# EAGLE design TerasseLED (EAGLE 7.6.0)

## Sheet 1 of 4: Spannungsversorgung + Controller + DALI
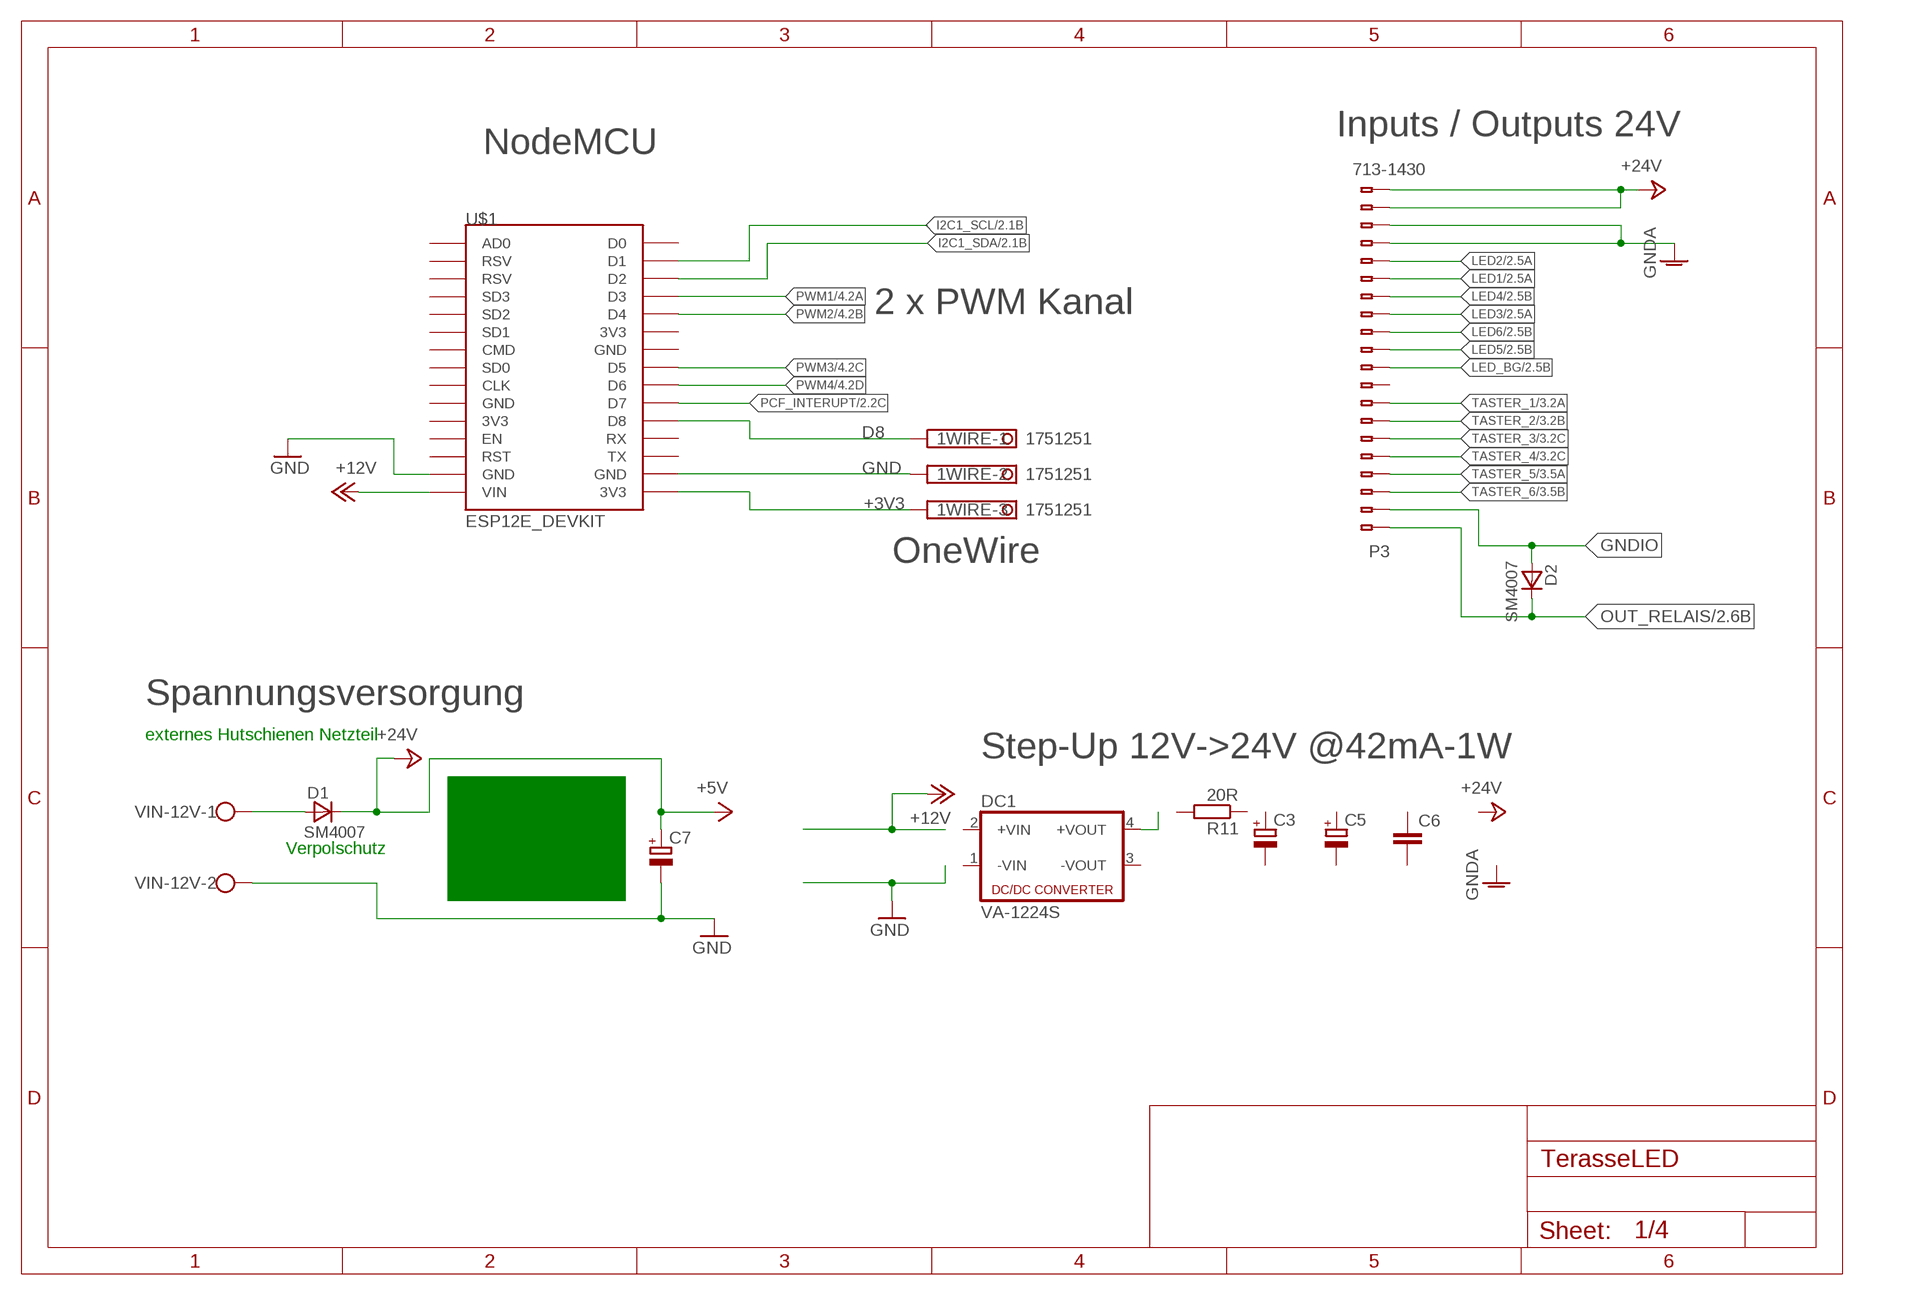
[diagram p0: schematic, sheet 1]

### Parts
1WIRE  1751251  [1751251]
C3  CPOL-EU140CLH-0810  [140CLH-0810]
C5  CPOL-EU140CLH-0810  [140CLH-0810]
C6  C-EUC0805  [C0805]
C7  CPOL-EU140CLH-0810  [140CLH-0810]
D1  SM4007  [MELF-MLL41]
D2  SM4007  [MELF-MLL41]
DC1  VA-1224S  [4SIL]
P3  713-1430  [713-1425]
R11  20R  R-EU_R1206  [R1206]
U$1  ESP12E_DEVKIT  [ESP12E_DEVKIT]
VIN-12V  W237-102  [W237-102]

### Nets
+3V3: 1WIRE.3 U$1.3V3@2(3V3) ; also sheet 2,3
+12V: U$1.VIN
+24V: C7.+ D1.C P3.19(B-19) P3.20(B-20) ; supply symbol labelled +5V ; also sheet 2
D8: 1WIRE.1 U$1.D8
GND: 1WIRE.2 C7.- U$1.GND@1(GND) U$1.GND@3(GND) VIN-12V.2 ; also sheet 2,3,4
GNDA: P3.17(B-17) P3.18(B-18) ; also sheet 2
GNDIO: D2.A P3.2(B-2) ; also sheet 2,3
I2C1_SCL: U$1.D1 ; also sheet 2
I2C1_SDA: U$1.D2 ; also sheet 2
LED1: P3.15(B-15) ; also sheet 2
LED2: P3.16(B-16) ; also sheet 2
LED3: P3.13(B-13) ; also sheet 2
LED4: P3.14(B-14) ; also sheet 2
LED5: P3.11(B-11) ; also sheet 2
LED6: P3.12(B-12) ; also sheet 2
LED_BG: P3.10(B-10) ; also sheet 2
N$1: D1.A VIN-12V.1
N$2: DC1.4(+VOUT)
OUT_RELAIS: D2.C P3.1(B-1) ; also sheet 2
PCF_INTERUPT: U$1.D7 ; also sheet 2
PWM1: U$1.D3 ; also sheet 4
PWM2: U$1.D4 ; also sheet 4
PWM3: U$1.D5 ; also sheet 4
PWM4: U$1.D6 ; also sheet 4
TASTER_1: P3.8(B-8) ; also sheet 3
TASTER_2: P3.7(B-7) ; also sheet 3
TASTER_3: P3.6(B-6) ; also sheet 3
TASTER_4: P3.5(B-5) ; also sheet 3
TASTER_5: P3.4(B-4) ; also sheet 3
TASTER_6: P3.3(B-3) ; also sheet 3
Unconnected: C3.+ C3.- C5.+ C5.- C6.1 C6.2 DC1.1(-VIN) DC1.2(+VIN) DC1.3(-VOUT) P3.9(B-9) R11.1 R11.2 U$1.3V3@0(3V3) U$1.3V3@1(3V3) U$1.AD0 U$1.CLK U$1.CMD U$1.D0 U$1.EN U$1.GND@0(GND) U$1.GND@2(GND) U$1.RST U$1.RSV@0(RSV) U$1.RSV@1(RSV) U$1.RX U$1.SD0 U$1.SD1 U$1.SD2 U$1.SD3 U$1.TX

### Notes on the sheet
- Inputs / Outputs 24V
- NodeMCU
- 2 x PWM Kanal
- OneWire
- Spannungsversorgung
- externes Hutschienen Netzteil
- Step-Up 12V->24V @42mA-1W
- Verpolschutz

## Sheet 2 of 4: Inputs & Outputs
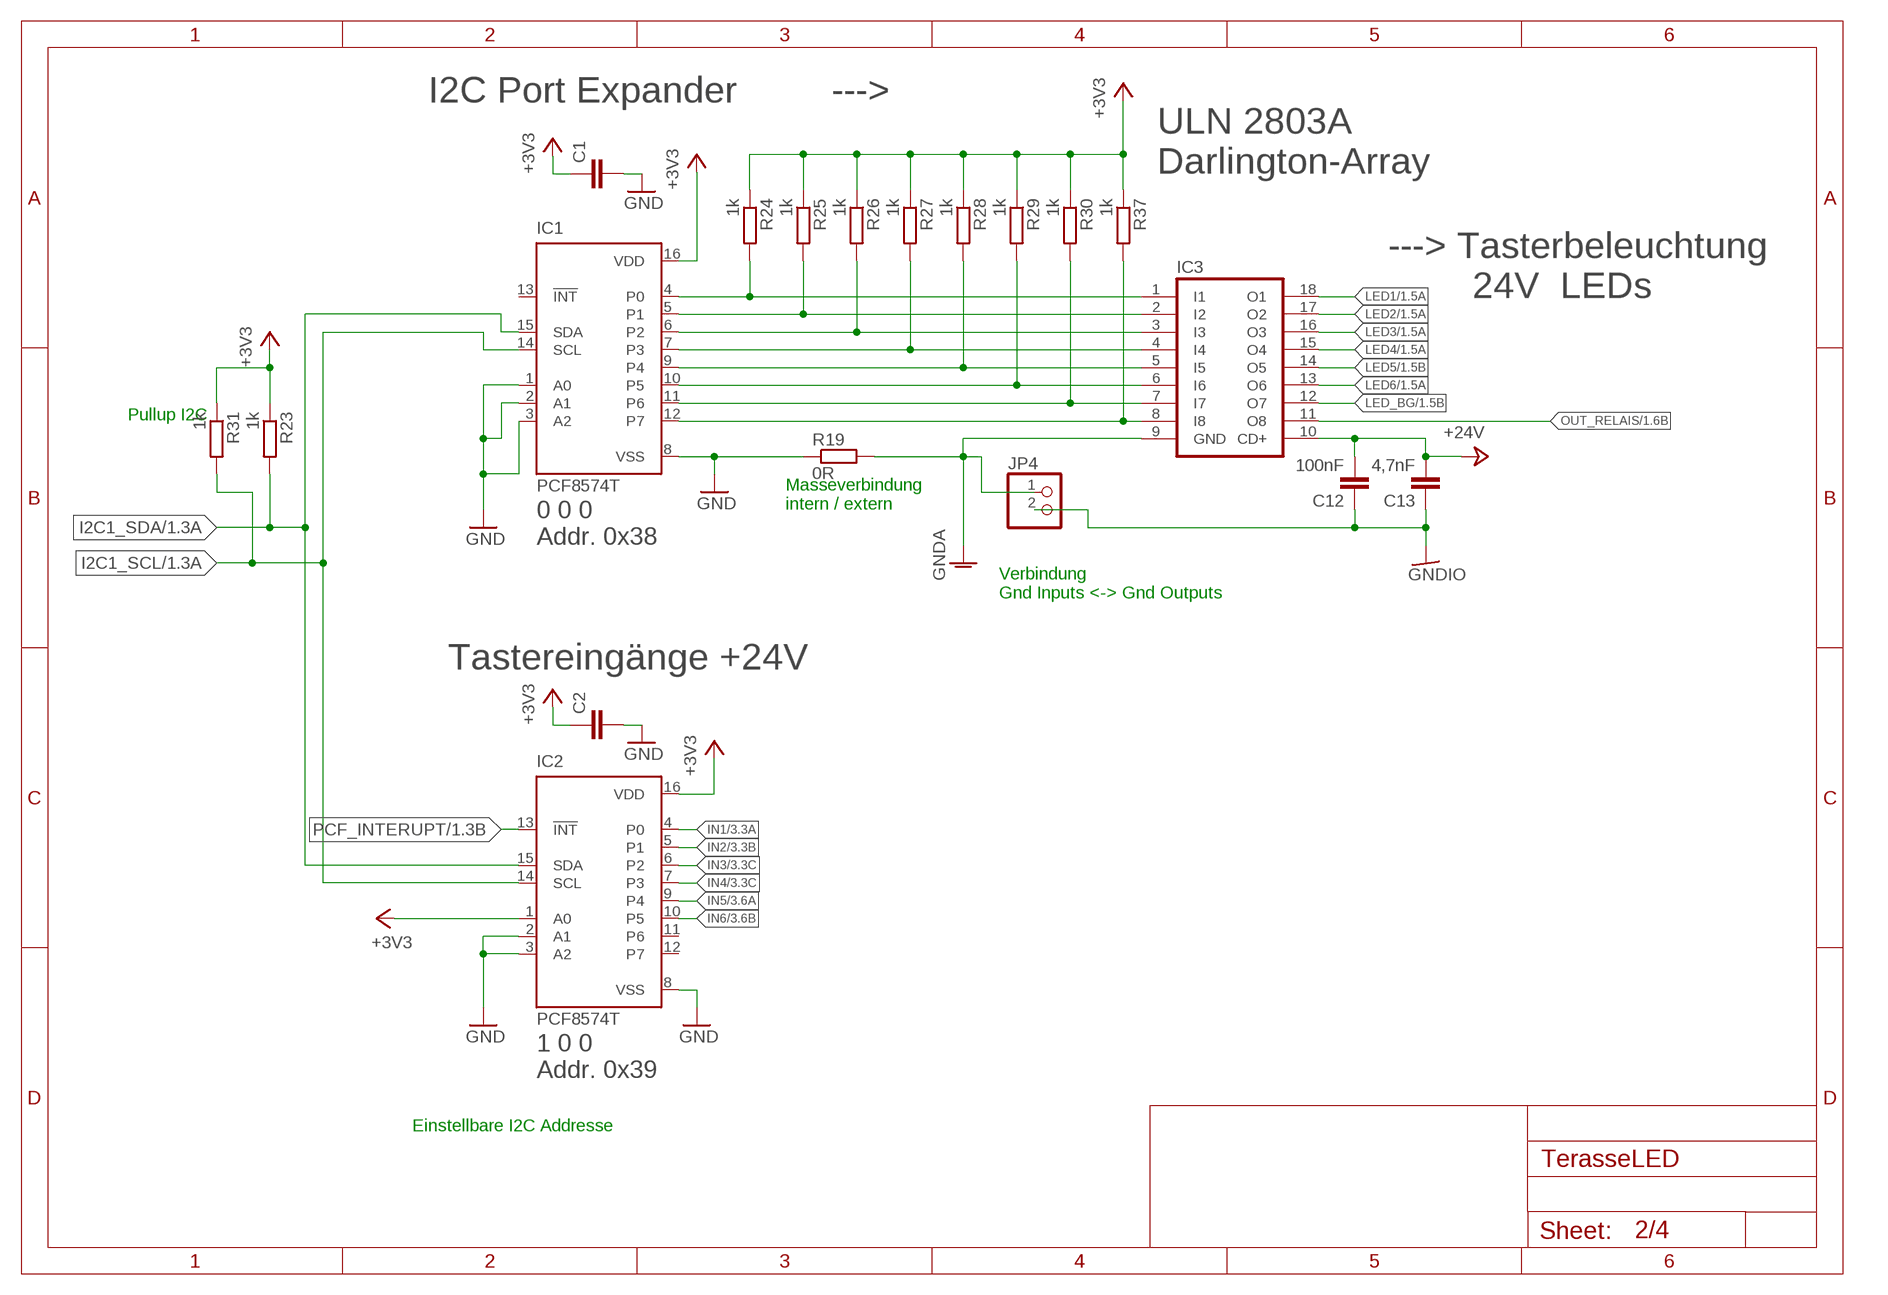
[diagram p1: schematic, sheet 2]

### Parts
C1  C-EUC0805  [C0805]
C2  C-EUC0805  [C0805]
C12  100nF  C-EUC0805  [C0805]
C13  4,7nF  C-EUC0805  [C0805]
IC1  PCF8574T  [SO16W]
IC2  PCF8574T  [SO16W]
IC3  ULN2803ASOP18  [SOP18]
JP4  PINHD-1X2  [1X02]
R19  0R  R-EU_R0805  [R0805]
R23  1k  R-EU_R0805  [R0805]
R24  1k  R-EU_R0805  [R0805]
R25  1k  R-EU_R0805  [R0805]
R26  1k  R-EU_R0805  [R0805]
R27  1k  R-EU_R0805  [R0805]
R28  1k  R-EU_R0805  [R0805]
R29  1k  R-EU_R0805  [R0805]
R30  1k  R-EU_R0805  [R0805]
R31  1k  R-EU_R0805  [R0805]
R37  1k  R-EU_R0805  [R0805]

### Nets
+3V3: C1.1 C2.1 IC1.16(VDD) IC2.1(A0) IC2.16(VDD) R23.1 R24.1 R25.1 R26.1 R27.1 R28.1 R29.1 R30.1 R31.1 R37.1 ; also sheet 1,3
+24V: C12.2 C13.2 IC3.10(CD+) ; also sheet 1
GND: C1.2 C2.2 IC1.1(A0) IC1.2(A1) IC1.3(A2) IC1.8(VSS) IC2.2(A1) IC2.3(A2) IC2.8(VSS) R19.1 ; also sheet 1,3,4
GNDA: IC3.9(GND) JP4.1 R19.2 ; also sheet 1
GNDIO: C12.1 C13.1 JP4.2 ; also sheet 1,3
I2C1_SCL: IC1.14(SCL) IC2.14(SCL) R31.2 ; also sheet 1
I2C1_SDA: IC1.15(SDA) IC2.15(SDA) R23.2 ; also sheet 1
IC1_P0: IC1.4(P0) IC3.1(I1) R24.2
IC1_P1: IC1.5(P1) IC3.2(I2) R25.2
IC1_P2: IC1.6(P2) IC3.3(I3) R26.2
IC1_P3: IC1.7(P3) IC3.4(I4) R27.2
IC1_P4: IC1.9(P4) IC3.5(I5) R28.2
IC1_P5: IC1.10(P5) IC3.6(I6) R29.2
IC1_P6: IC1.11(P6) IC3.7(I7) R30.2
IN1: IC2.4(P0) ; also sheet 3
IN2: IC2.5(P1) ; also sheet 3
IN3: IC2.6(P2) ; also sheet 3
IN4: IC2.7(P3) ; also sheet 3
IN5: IC2.9(P4) ; also sheet 3
IN6: IC2.10(P5) ; also sheet 3
LED1: IC3.18(O1) ; also sheet 1
LED2: IC3.17(O2) ; also sheet 1
LED3: IC3.16(O3) ; also sheet 1
LED4: IC3.15(O4) ; also sheet 1
LED5: IC3.14(O5) ; also sheet 1
LED6: IC3.13(O6) ; also sheet 1
LED_BG: IC3.12(O7) ; also sheet 1
N$19: IC1.12(P7) IC3.8(I8) R37.2
OUT_RELAIS: IC3.11(O8) ; also sheet 1
PCF_INTERUPT: IC2.13(!INT) ; also sheet 1
Unconnected: IC1.13(!INT) IC2.11(P6) IC2.12(P7)

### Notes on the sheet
- I2C Port Expander         --->
- ULN 2803A 
  Darlington-Array
- ---> Tasterbeleuchtung 
          24V  LEDs
- Pullup I2C
- Masseverbindung
  intern / extern
- 0 0 0 
  Addr. 0x38
- Verbindung 
  Gnd Inputs <-> Gnd Outputs
- Tastereingänge +24V
- 1 0 0 
  Addr. 0x39
- Einstellbare I2C Addresse

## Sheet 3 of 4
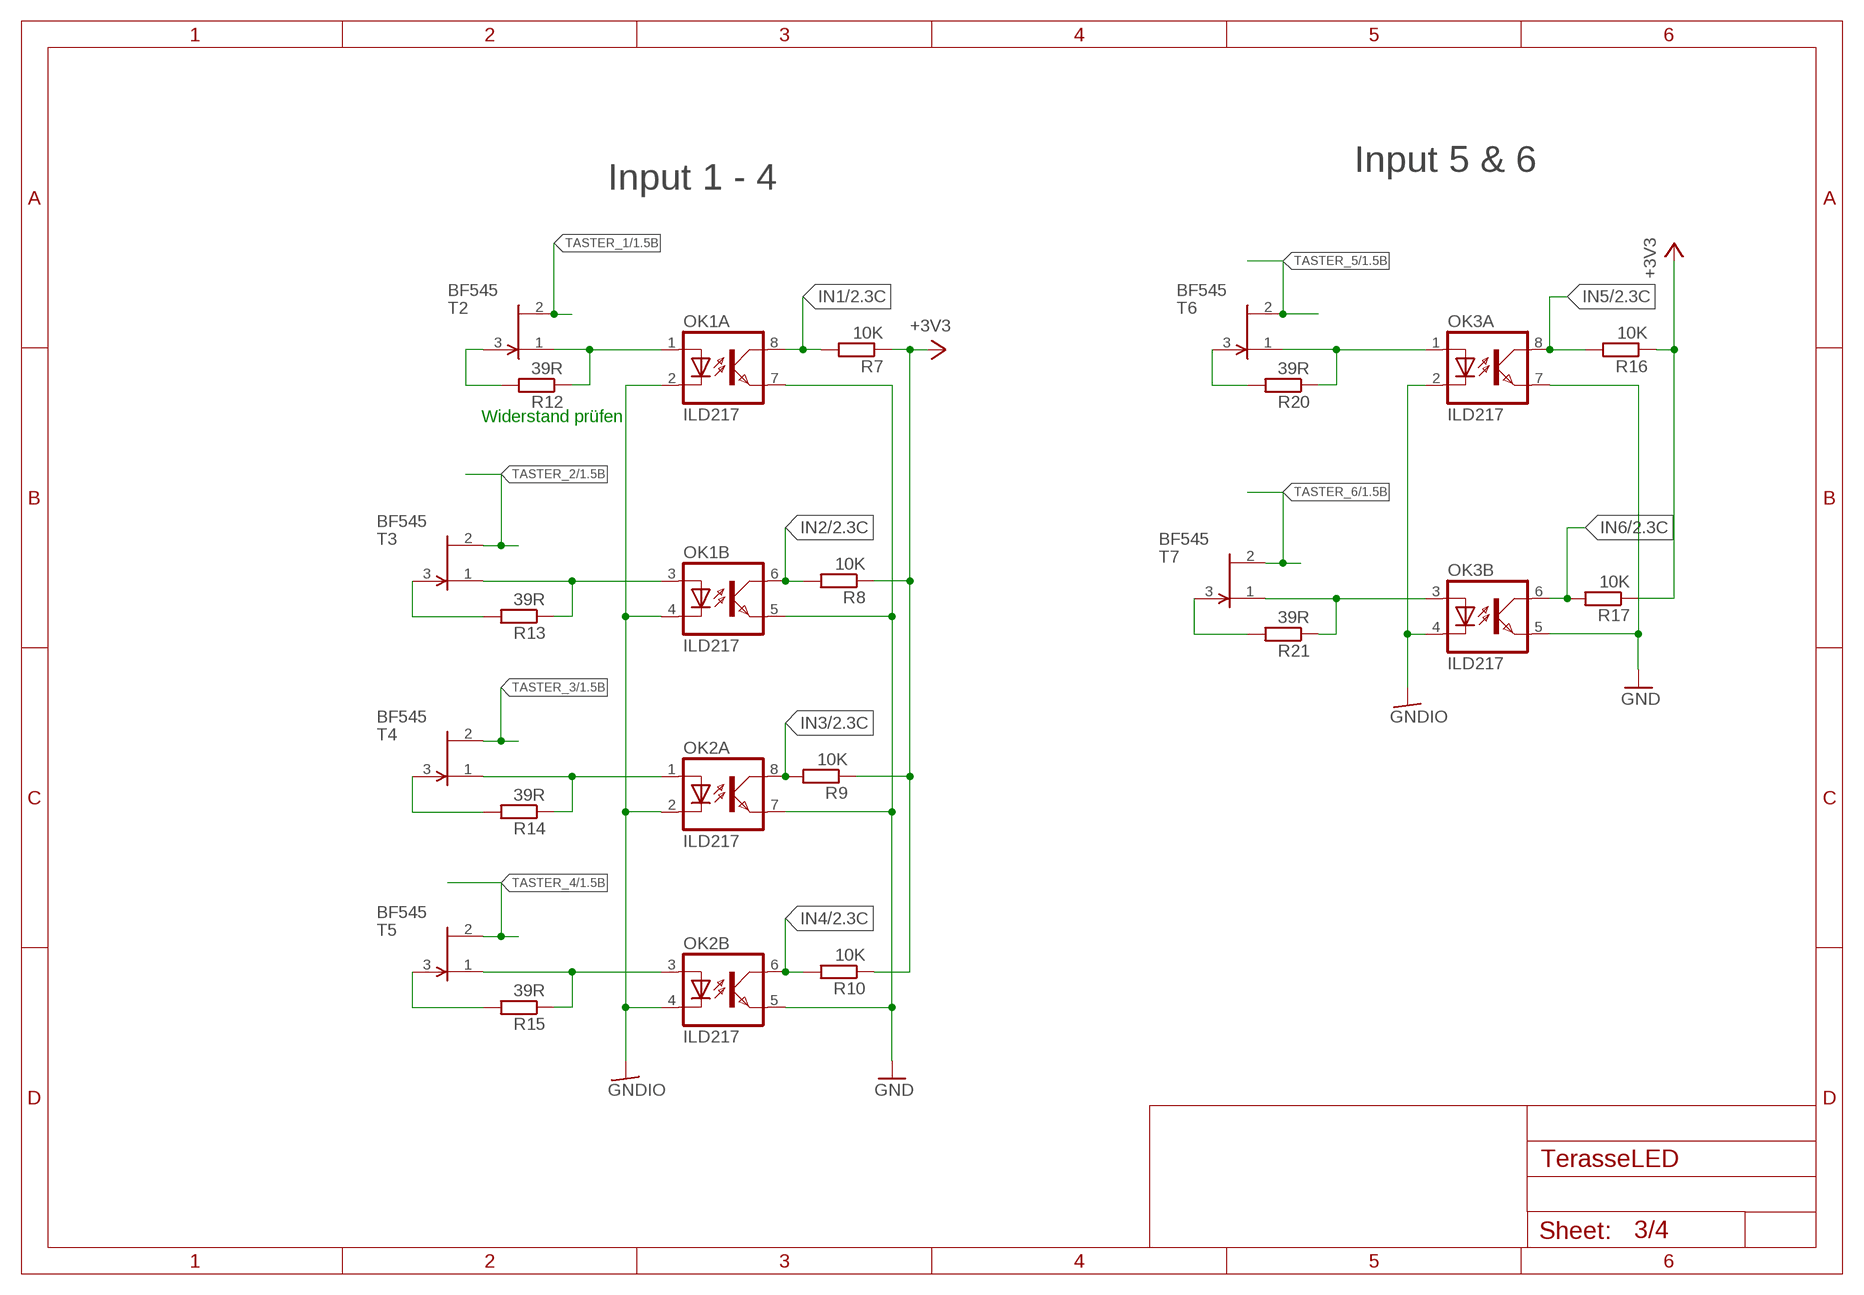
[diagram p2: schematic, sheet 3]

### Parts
OK1  ILD217  [SOIC08]
OK2  ILD217  [SOIC08]
OK3  ILD217  [SOIC08]
R7  10K  R-EU_R0805  [R0805]
R8  10K  R-EU_R0805  [R0805]
R9  10K  R-EU_R0805  [R0805]
R10  10K  R-EU_R0805  [R0805]
R12  39R  R-EU_R0805  [R0805]
R13  39R  R-EU_R0805  [R0805]
R14  39R  R-EU_R0805  [R0805]
R15  39R  R-EU_R0805  [R0805]
R16  10K  R-EU_R0805  [R0805]
R17  10K  R-EU_R0805  [R0805]
R20  39R  R-EU_R0805  [R0805]
R21  39R  R-EU_R0805  [R0805]
T2  BF545  [SOT23]
T3  BF545  [SOT23]
T4  BF545  [SOT23]
T5  BF545  [SOT23]
T6  BF545  [SOT23]
T7  BF545  [SOT23]

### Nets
+3V3: R7.1 R8.1 R9.1 R10.1 R16.1 R17.1 ; also sheet 1,2
GND: OK1.5(B:EMIT) OK1.7(A:EMIT) OK2.5(B:EMIT) OK2.7(A:EMIT) OK3.5(B:EMIT) OK3.7(A:EMIT) ; also sheet 1,2,4
GNDIO: OK1.2(A:C) OK1.4(B:C) OK2.2(A:C) OK2.4(B:C) OK3.2(A:C) OK3.4(B:C) ; also sheet 1,2
IN1: OK1.8(A:COL) R7.2 ; also sheet 2
IN2: OK1.6(B:COL) R8.2 ; also sheet 2
IN3: OK2.8(A:COL) R9.2 ; also sheet 2
IN4: OK2.6(B:COL) R10.2 ; also sheet 2
IN5: OK3.8(A:COL) R16.2 ; also sheet 2
IN6: OK3.6(B:COL) R17.2 ; also sheet 2
N$3: OK2.3(B:A) R15.1 T5.1(S)
N$7: OK2.1(A:A) R14.1 T4.1(S)
N$8: OK1.3(B:A) R13.1 T3.1(S)
N$10: R13.2 T3.3(G)
N$11: R14.2 T4.3(G)
N$12: R15.2 T5.3(G)
N$13: R12.2 T2.3(G)
N$16: OK3.3(B:A) R21.1 T7.1(S)
N$17: R21.2 T7.3(G)
N$20: R20.2 T6.3(G)
Q9_P0_IN: OK1.1(A:A) R12.1 T2.1(S)
Q9_P0_IN1: OK3.1(A:A) R20.1 T6.1(S)
TASTER_1: T2.2(D) ; also sheet 1
TASTER_2: T3.2(D) ; also sheet 1
TASTER_3: T4.2(D) ; also sheet 1
TASTER_4: T5.2(D) ; also sheet 1
TASTER_5: T6.2(D) ; also sheet 1
TASTER_6: T7.2(D) ; also sheet 1

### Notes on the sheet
- Input 5 & 6
- Input 1 - 4
- Widerstand prüfen

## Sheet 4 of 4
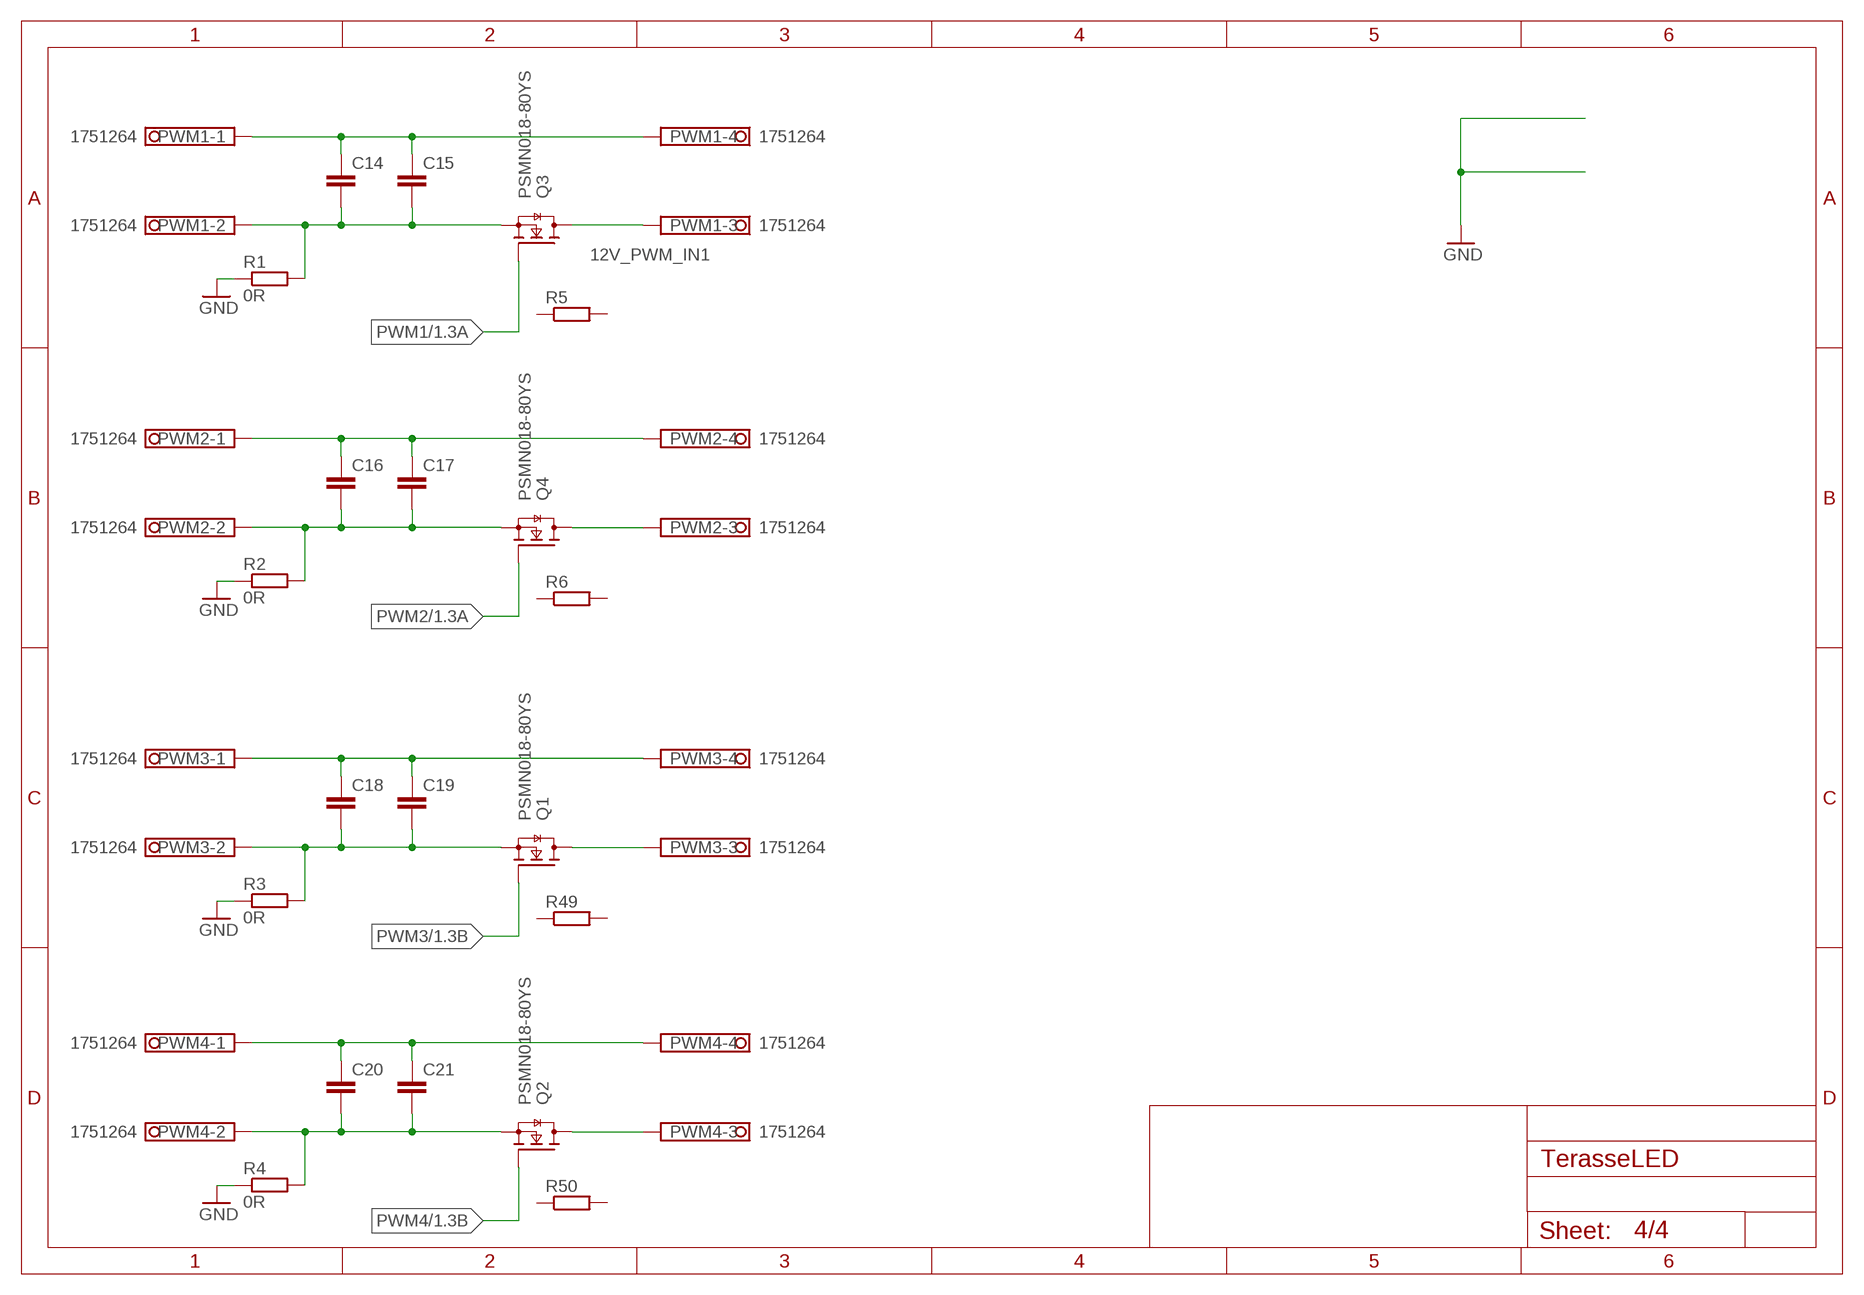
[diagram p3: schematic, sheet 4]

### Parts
C14  C-EUC1206  [C1206]
C15  C-EUC1206  [C1206]
C16  C-EUC1206  [C1206]
C17  C-EUC1206  [C1206]
C18  C-EUC1206  [C1206]
C19  C-EUC1206  [C1206]
C20  C-EUC1206  [C1206]
C21  C-EUC1206  [C1206]
PWM1  1751264  [1751264]
PWM2  1751264  [1751264]
PWM3  1751264  [1751264]
PWM4  1751264  [1751264]
Q1  PSMN018-80YS  [SOT669]
Q2  PSMN018-80YS  [SOT669]
Q3  PSMN018-80YS  [SOT669]
Q4  PSMN018-80YS  [SOT669]
R1  0R  R-EU_R0603  [R0603]
R2  0R  R-EU_R0603  [R0603]
R3  0R  R-EU_R0603  [R0603]
R4  0R  R-EU_R0603  [R0603]
R5  R-EU_R0805  [R0805]
R6  R-EU_R0805  [R0805]
R49  R-EU_R0805  [R0805]
R50  R-EU_R0805  [R0805]

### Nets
12V_PWM_IN1: PWM1.3 Q3.MB(D)
GND: R1.1 R2.1 R3.1 R4.1 ; also sheet 1,2,3
N$4: C14.2 C15.2 PWM1.2 Q3.1(S) Q3.2(S) Q3.3(S) R1.2
N$5: C16.2 C17.2 PWM2.2 Q4.1(S) Q4.2(S) Q4.3(S) R2.2
N$6: C14.1 C15.1 PWM1.1 PWM1.4
N$9: C16.1 C17.1 PWM2.1 PWM2.4
N$21: PWM3.3 Q1.MB(D)
N$25: C18.2 C19.2 PWM3.2 Q1.1(S) Q1.2(S) Q1.3(S) R3.2
N$26: PWM2.3 Q4.MB(D)
N$27: C18.1 C19.1 PWM3.1 PWM3.4
N$28: PWM4.3 Q2.MB(D)
N$29: C20.2 C21.2 PWM4.2 Q2.1(S) Q2.2(S) Q2.3(S) R4.2
N$30: C20.1 C21.1 PWM4.1 PWM4.4
PWM1: Q3.4(G) ; also sheet 1
PWM2: Q4.4(G) ; also sheet 1
PWM3: Q1.4(G) ; also sheet 1
PWM4: Q2.4(G) ; also sheet 1
Unconnected: R5.1 R5.2 R6.1 R6.2 R49.1 R49.2 R50.1 R50.2

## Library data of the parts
1WIRE = con-phoenix-350:1751251: MKDS 1/ 3-3,5 Printklemme Nennstrom: 10 A Bemessungsspannung: 160 V Raster: 3,5 mm Polzahl: 3 Montageart: Löten Anschlussart: Schraubanschluss Anschlussrichtung vom Leiter zur Platine: 0° Source: http://eshop.phoenixcontact.com .. 1751251.pdf; OC_FARNELL: unknown; OC_NEWARK: unknown
C1 C2 C12 C13 = rcl:C-EU: CAPACITOR, European symbol
C3 C5 C7 = resistor:CPOL-EU: POLARIZED CAPACITOR, European symbol
C6 C14-C21 = resistor:C-EU: CAPACITOR, European symbol
D1 D2 = _mod_diode:SM400*: SM4001 .. SM4007 General Purpose Rectifier, 1 A
DC1 = dc-dc-converter:VA-*?: DC DC Converter Single Output, 1 Watt Motien Technology Co.,Ltd. Source: va-serie.pdf
IC1 IC2 = micro-philips:PCF8574: I2C-Bus Remote 8-bit I/O expander http://www.semiconductors.philips.com/acrobat_download/datasheets/PCF8574_4.pdf; MPN: PCF8574T/3,512; OC_FARNELL: 1201255; OC_NEWARK: 70R6870
IC3 = uln-udn:ULN2803A: DRIVER ARRAY
JP4 = pinhead:PINHD-1X2: PIN HEADER
OK1-OK3 = optocoupler:ILD2*: Siemens ILD205/206/207/211/213/217 DUAL PHOTOTRANSISTOR SMALL OUTLINE SURFACE MOUNT OPTOCOUPLER Source: 153385-da-01-en-Optocoupler_ILD205-T.pdf; MF: VISHAY/TELEFUNKEN; MPN: ILD217T; OC_FARNELL: 1469515RL; OC_NEWARK: 20H8681
P3 = con-wago255:713-1430
PWM1-PWM4 = con-phoenix-350:1751264: MKDS 1/ 4-3,5 Printklemme Nennstrom: 10 A Bemessungsspannung: 160 V Raster: 3,5 mm Polzahl: 4 Montageart: Löten Anschlussart: Schraubanschluss Anschlussrichtung vom Leiter zur Platine: 0° Source: http://eshop.phoenixcontact.com .. 1751264.pdf; MPN: 1751264; OC_FARNELL: unknown; OC_NEWARK: 10R0934
Q1-Q4 = NXP_60_26022015:PSMN: N-channel logic level TrenchMOS(TM) transistor AAL Eindhoven MK
R1-R6 R11 R19 R37 R49 R50 = resistor:R-EU_: RESISTOR, European symbol
R7-R10 R12-R17 R20 R21 R23-R31 = rcl:R-EU_: RESISTOR, European symbol
T2-T7 = NXP_60_26022015:BF545
U$1 = ESP12E_DEVKIT:ESP12E_DEVKIT: ESP12E DEVKIT BOARD
VIN-12V = con-wago-500:W237-102: WAGO SCREW CLAMP; MPN: 237-102; OC_FARNELL: unknown; OC_NEWARK: 70K9898

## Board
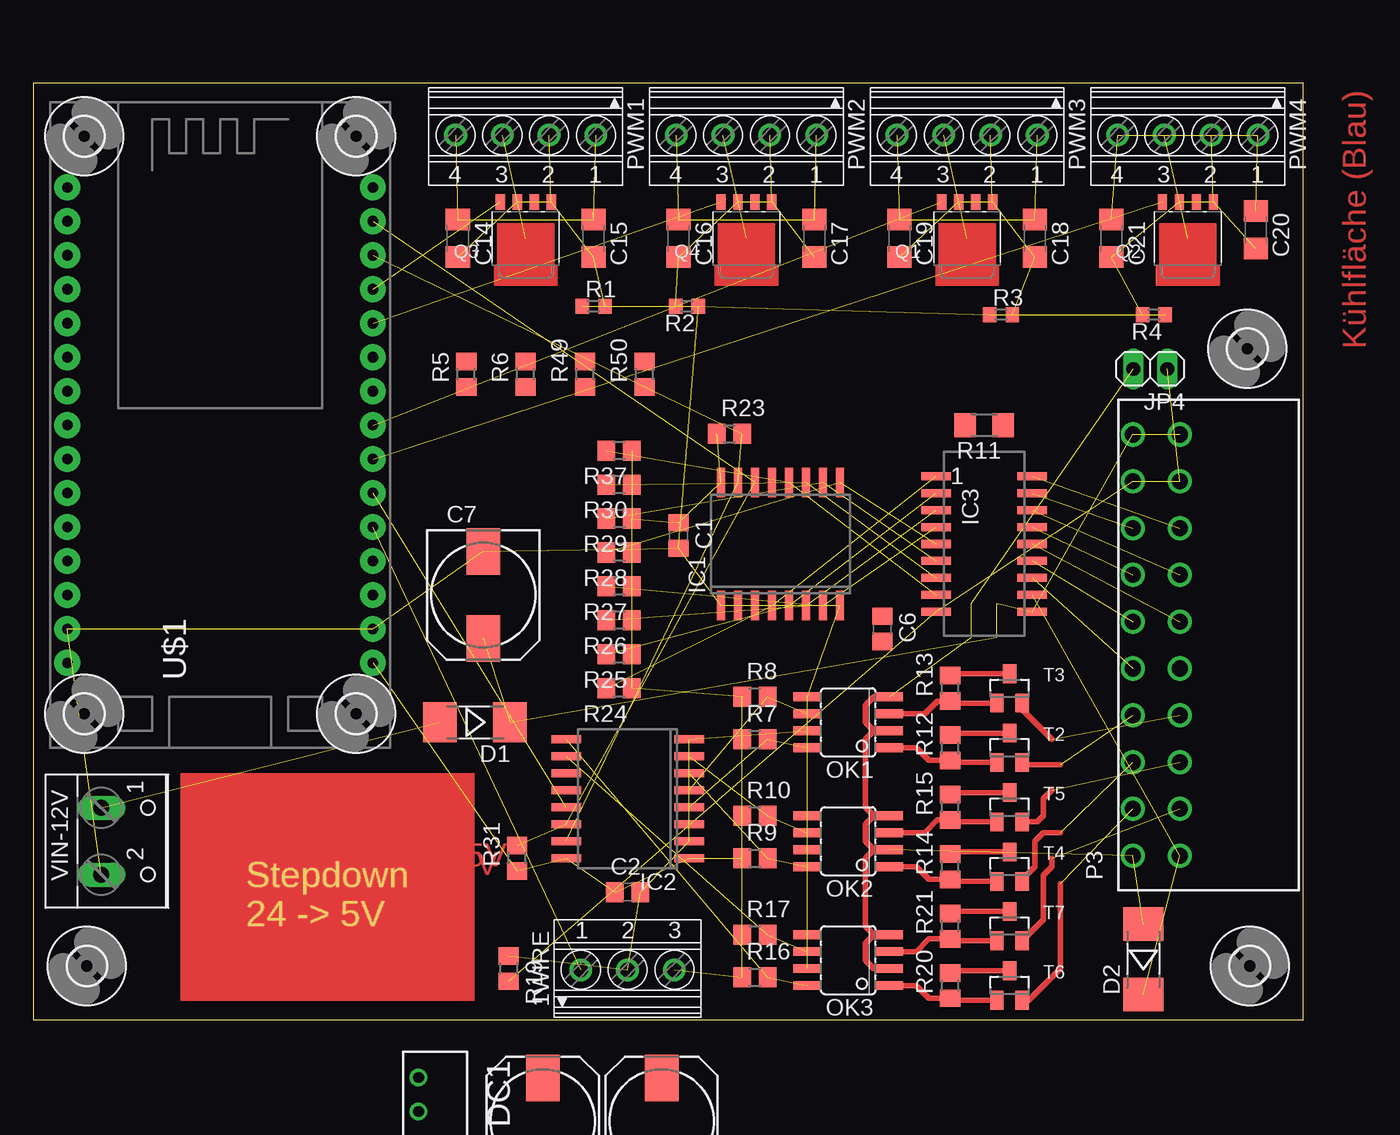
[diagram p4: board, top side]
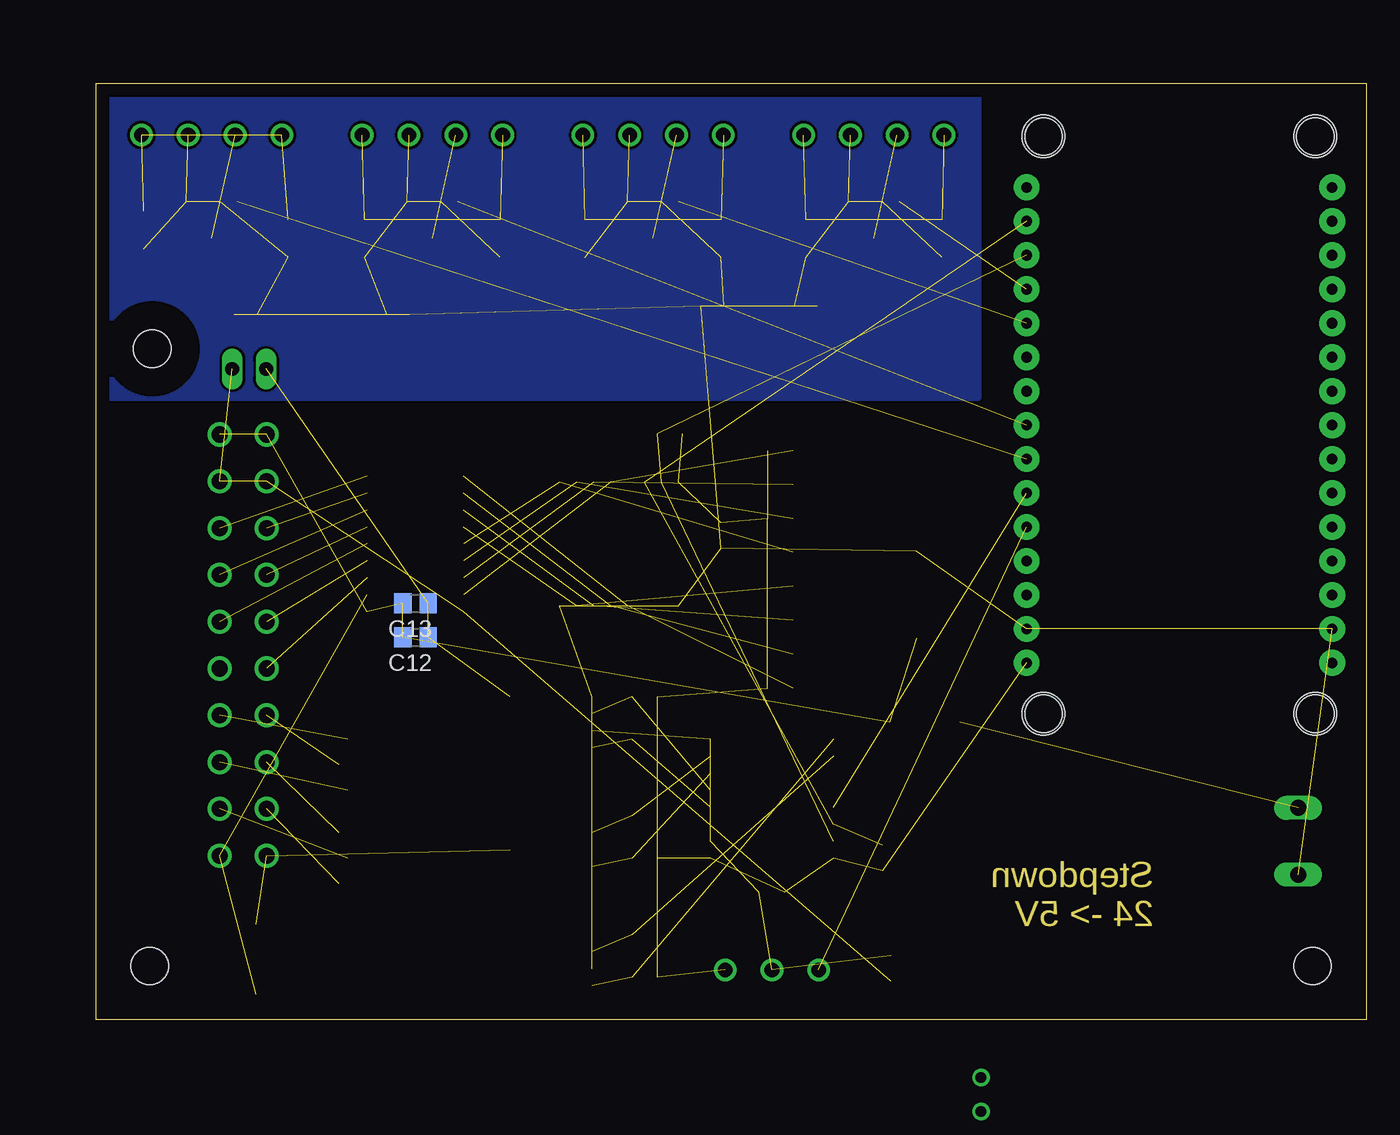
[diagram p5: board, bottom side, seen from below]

Size 95 x 70 mm. Coordinates in mm from the lower left corner, seen from the top.
Outline: 95,0 95,70 0,70 0,0 95,0
Copper layers (1*16): Top 0.035mm / dielectric 1.5mm / Bottom 0.035mm
Design rules "default": minimum track width 10mil, minimum drill 24mil, track to track 8mil, track to pad 8mil, pad to pad 8mil, via to via 8mil, smd to smd 8mil, copper to edge 40mil, drill to drill 8mil, minimum pad ring 10mil, minimum via ring 8mil, stop-mask expansion 4mil, vias tented up to drill 0mil, thermal gap 10mil

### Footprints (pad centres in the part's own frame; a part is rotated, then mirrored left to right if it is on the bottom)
1751251 = drill 1.1 pad 1.7: 1 -3.5,-0.1; 2 0,-0.1; 3 3.5,-0.1
C0805 = smd 1.3 x 1.5: 1 -0.95,0; 2 0.95,0
140CLH-0810 = smd 3.5 x 2.5: + 3.25,0; - -3.25,0
C1206 = smd 1.6 x 1.8: 1 -1.4,0; 2 1.4,0
MELF-MLL41 = smd 2.5 x 3: A 2.625,0; C -2.625,0
4SIL = drill 0.8: 1 -3.81,0; 2 -1.27,0; 3 1.27,0; 4 3.81,0
SO16W = smd 0.6 x 2.2: 1 -4.445,-4.6; 2 -3.175,-4.6; 3 -1.905,-4.6; 4 -0.635,-4.6; 5 0.635,-4.6; 6 1.905,-4.6; 7 3.175,-4.6; 8 4.445,-4.6; 9 4.445,4.6; 10 3.175,4.6; 11 1.905,4.6; 12 0.635,4.6; 13 -0.635,4.6; 14 -1.905,4.6; 15 -3.175,4.6; 16 -4.445,4.6
SOP18 = smd 0.6 x 2.2: 1 -5.08,-3.6; 2 -3.81,-3.6; 3 -2.54,-3.6; 4 -1.27,-3.6; 5 0,-3.6; 6 1.27,-3.6; 7 2.54,-3.6; 8 3.81,-3.6; 9 5.08,-3.6; 10 5.08,3.6; 11 3.81,3.6; 12 2.54,3.6; 13 1.27,3.6; 14 0,3.6; 15 -1.27,3.6; 16 -2.54,3.6; 17 -3.81,3.6; 18 -5.08,3.6
1X02 = drill 1.016 long: 1 -1.27,0; 2 1.27,0
SOIC08 = smd 0.66 x 2.032: 1 -1.905,-3.073; 2 -0.635,-3.073; 3 0.635,-3.073; 4 1.905,-3.073; 5 1.905,3.073; 6 0.635,3.073; 7 -0.635,3.073; 8 -1.905,3.073
713-1425 = drill 1.2: 1 -15.75,-1.75; 2 -15.75,1.75; 3 -12.25,-1.75; 4 -12.25,1.75; 5 -8.75,-1.75; 6 -8.75,1.75; 7 -5.25,-1.75; 8 -5.25,1.75; 9 -1.75,-1.75; 10 -1.75,1.75; 11 1.75,-1.75; 12 1.75,1.75; 13 5.25,-1.75; 14 5.25,1.75; 15 8.75,-1.75; 16 8.75,1.75; 17 12.25,-1.75; 18 12.25,1.75; 19 15.75,-1.75; 20 15.75,1.75
1751264 = drill 1.1 pad 1.7: 1 -5.25,-0.1; 2 -1.75,-0.1; 3 1.75,-0.1; 4 5.25,-0.1
SOT669 = smd 0.7 x 1.15: 1 -1.905,-2.725; 2 -0.636,-2.725; 3 0.635,-2.725; 4 1.905,-2.725 | smd 0 x 0: MB 0,0
R0603 = smd 1 x 1.1: 1 -0.85,0; 2 0.85,0
R0805 = smd 1.3 x 1.5: 1 -0.95,0; 2 0.95,0
R1206 = smd 1.6 x 1.803: 1 -1.422,0; 2 1.422,0
SOT23 = smd 1 x 1.4: 1 -0.95,-1.1; 2 0.95,-1.1; 3 0,1.1
ESP12E_DEVKIT = drill 0.8 pad 1.93: 3V3@0 -11.43,-7.62; 3V3@1 11.43,5.08; 3V3@2 11.43,-17.78; AD0 -11.43,17.78; CLK -11.43,-2.54; CMD -11.43,2.54; D0 11.43,17.78; D1 11.43,15.24; D2 11.43,12.7; D3 11.43,10.16; D4 11.43,7.62; D5 11.43,0; D6 11.43,-2.54; D7 11.43,-5.08; D8 11.43,-7.62; EN -11.43,-10.16; GND@0 -11.43,-5.08; GND@1 -11.43,-15.24; GND@2 11.43,2.54; GND@3 11.43,-15.24; RST -11.43,-12.7; RSV@0 -11.43,15.24; RSV@1 -11.43,12.7; RX 11.43,-10.16; SD0 -11.43,0; SD1 -11.43,5.08; SD2 -11.43,7.62; SD3 -11.43,10.16; TX 11.43,-12.7; VIN -11.43,-17.78 | hole 3.2: -10.16,21.59; 10.16,21.59; 10.16,-21.59; -10.16,-21.59
2,8 = hole 2.8: 0,0
W237-102 = drill 1.194 long: 1 -2.5,-1.27; 2 2.5,-1.27

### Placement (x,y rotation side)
1WIRE  44.45,3.81 0 top
C1  48.26,36.2 270 top
C2  44.45,9.53 0 top
C3  not placed on the board
C5  not placed on the board
C6  63.5,29.21 270 top
C7  33.66,31.75 270 top
C12  71.12,28.57 180 bottom
C13  71.12,31.11 180 bottom
C14  31.75,58.42 270 top
C15  41.91,58.42 270 top
C16  48.26,58.42 270 top
C17  58.42,58.42 270 top
C18  74.93,58.42 270 top
C19  64.77,58.42 270 top
C20  91.44,59.05 270 top
C21  80.64,58.42 270 top
D1  33.02,22.23 180 top
D2  83.03,4.51 90 top
DC1  not placed on the board
IC1  55.88,35.56 0 top
IC2  44.45,16.51 90 top
IC3  71.12,35.56 270 top
JP4  83.56,48.65 180 top
OK1  60.96,22.23 90 top
OK2  60.96,13.34 90 top
OK3  60.96,4.45 90 top
P3  84,28 90 top
PWM1  36.83,66.04 180 top
PWM2  53.34,66.04 180 top
PWM3  69.85,66.04 180 top
PWM4  86.36,66.04 180 top
Q1  69.85,58.42 180 top
Q2  86.36,58.42 180 top
Q3  36.83,58.42 180 top
Q4  53.34,58.42 180 top
R1  41.91,53.34 0 top
R2  48.9,53.34 180 top
R3  72.39,52.7 0 top
R4  83.82,52.7 180 top
R5  32.38,48.26 90 top
R6  36.83,48.26 90 top
R7  53.98,20.95 0 top
R8  53.98,24.13 0 top
R9  53.98,12.06 0 top
R10  53.98,15.24 0 top
R11  71.12,44.45 180 top
R12  68.58,20.32 90 top
R13  68.58,24.77 90 top
R14  68.58,11.43 90 top
R15  68.58,15.88 90 top
R16  53.98,3.17 0 top
R17  53.98,6.35 0 top
R19  35.56,3.81 270 top
R20  68.58,2.54 90 top
R21  68.58,6.99 90 top
R23  52.07,43.81 0 top
R24  43.81,24.77 180 top
R25  43.81,27.3 180 top
R26  43.81,29.84 180 top
R27  43.81,32.38 180 top
R28  43.81,34.92 180 top
R29  43.81,37.47 180 top
R30  43.81,40.01 180 top
R31  36.2,12.06 90 top
R37  43.81,42.55 180 top
R49  41.27,48.26 90 top
R50  45.72,48.26 90 top
T2  73.03,20.32 0 top
T3  73.03,24.77 0 top
T4  73.03,11.43 0 top
T5  73.03,15.88 0 top
T6  73.03,2.54 0 top
T7  73.03,6.99 0 top
U$1  13.97,44.45 0 top
U$2  [2,8]  3.81,66.04 0 top
U$3  [2,8]  3.81,22.86 0 top
U$4  [2,8]  24.13,22.86 0 top
U$5  [2,8]  24.13,66.04 0 top
U$6  [2,8]  90.81,50.16 0 top
U$7  [2,8]  4,4 0 top
U$8  [2,8]  91,4 0 top
VIN-12V  6.35,13.34 270 top

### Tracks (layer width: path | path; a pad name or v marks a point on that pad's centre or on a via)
12V_PWM_IN1  (1 unrouted)
+3V3  (22 unrouted)
+24V  (6 unrouted)
D8  (1 unrouted)
GND  (24 unrouted)
  pour Bottom: 29,46.46 29,69.5 95,69.5 95,46.46
GNDA  (4 unrouted)
GNDIO  (5 unrouted)
  Top 0.406: OK1.4 62.87,24.13 62.23,23.5 62.23,22.23 62.87,21.59 | OK1.2 62.87,21.59 | 62.87,21.59 62.23,20.95 62.23,15.88 62.87,15.24 | OK2.4 62.87,15.24 | 62.87,15.24 62.23,14.61 62.23,13.34 62.87,12.7 | 62.87,12.7 OK2.2 | 62.87,6.35 62.23,6.99 62.23,12.06 62.87,12.7 | OK3.4 62.87,6.35 | 62.87,6.35 62.23,5.71 62.23,4.45 62.87,3.81 OK3.2
I2C1_SCL  (3 unrouted)
I2C1_SDA  (3 unrouted)
IC1_P0  (2 unrouted)
IC1_P1  (2 unrouted)
IC1_P2  (2 unrouted)
IC1_P3  (2 unrouted)
IC1_P4  (2 unrouted)
IC1_P5  (2 unrouted)
IC1_P6  (2 unrouted)
IN1  (2 unrouted)
IN2  (2 unrouted)
IN3  (2 unrouted)
IN4  (2 unrouted)
IN5  (2 unrouted)
IN6  (2 unrouted)
LED1  (1 unrouted)
LED2  (1 unrouted)
LED3  (1 unrouted)
LED4  (1 unrouted)
LED5  (1 unrouted)
LED6  (1 unrouted)
LED_BG  (1 unrouted)
N$1  (1 unrouted)
N$3
  Top 0.406: T5.1 68.73,14.78 R15.1 67.63,14.93 66.67,13.97 OK2.3
N$4  (6 unrouted)
N$5  (6 unrouted)
N$6  (3 unrouted)
N$7
  Top 0.406: T4.1 68.73,10.33 R14.1 66.99,10.48 66.04,11.43 OK2.1
N$8
  Top 0.406: T3.1 68.73,23.66 R13.1 67.63,23.82 66.67,22.86 OK1.3
N$9  (3 unrouted)
N$10
  Top 0.406: T3.3 68.73,25.86 R13.2
N$11
  Top 0.406: T4.3 68.73,12.53 R14.2
N$12
  Top 0.406: T5.3 68.73,16.98 R15.2
N$13
  Top 0.406: T2.3 68.73,21.42 R12.2
N$16
  Top 0.406: T7.1 68.73,5.88 R21.1 67,6.04 66.04,5.08 OK3.3
N$17
  Top 0.406: T7.3 68.73,8.09 R21.2
N$19  (2 unrouted)
N$20
  Top 0.406: T6.3 68.73,3.64 R20.2
N$21  (1 unrouted)
N$25  (6 unrouted)
N$26  (1 unrouted)
N$27  (3 unrouted)
N$28  (1 unrouted)
N$29  (6 unrouted)
N$30  (3 unrouted)
OUT_RELAIS  (2 unrouted)
PCF_INTERUPT  (1 unrouted)
PWM1  (1 unrouted)
PWM2  (1 unrouted)
PWM3  (1 unrouted)
PWM4  (1 unrouted)
Q9_P0_IN
  Top 0.406: T2.1 68.73,19.22 R12.1 66.99,19.37 66.04,20.32 OK1.1
Q9_P0_IN1
  Top 0.406: T6.1 68.73,1.44 R20.1 66.99,1.59 66.04,2.54 OK3.1
TASTER_1  (1 unrouted)
  Top 0.406: 74.12,19.22 T2.2 74.14,19.05 76.83,19.05
TASTER_2  (1 unrouted)
  Top 0.406: T3.2 73.97,23.18 76.2,20.95
TASTER_3  (1 unrouted)
  Top 0.406: T4.2 73.97,10.47 74.93,11.43 74.93,13.34 75.56,13.97 76.83,13.97
TASTER_4  (1 unrouted)
  Top 0.406: T5.2 75.1,14.78 75.56,15.24 75.56,16.51 76.2,17.14
TASTER_5  (1 unrouted)
  Top 0.406: T6.2 74.47,1.44 76.83,3.81 76.83,10.16
TASTER_6  (1 unrouted)
  Top 0.406: 76.2,12.06 76.2,11.43 75.56,10.79 75.56,7.47 T7.2
(copper drawn outside any net)
  shapes: Top area x1

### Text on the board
Top: Kühlfläche (Blau) | Stepdown 24 -> 5V | Stepdown 24 -> 5V
Dimension: Stepdown / 24 -> 5V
